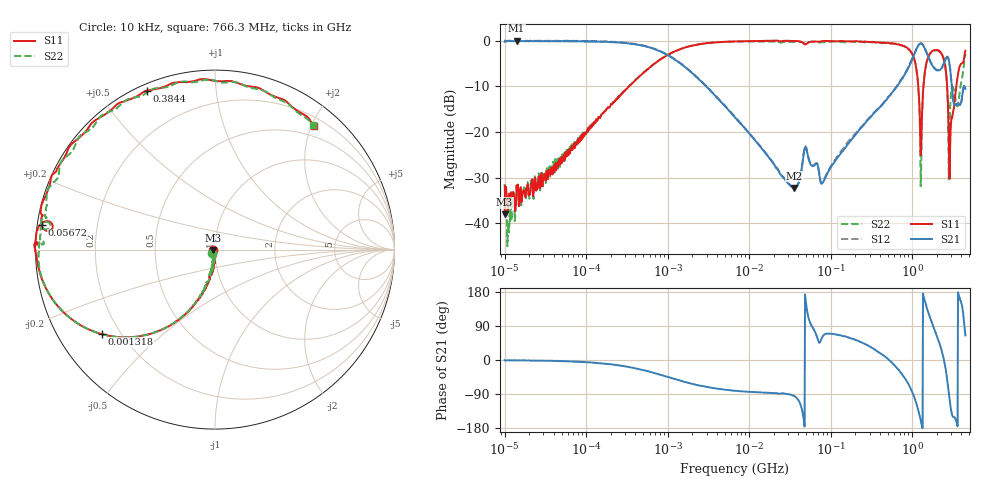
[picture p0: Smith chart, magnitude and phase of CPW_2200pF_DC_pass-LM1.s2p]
!Siglent Technologies,SNA5004A,SNA5XCED5R0097,V1.0.0.2.10.R9
!Date: 2024-10-29 17:12:58
!Data & Calibration Information:
!Freq	S11:F2(ON)	S21:F2(ON)	S12:F2(ON)	S22:F2(ON)
# Hz S DB R 50
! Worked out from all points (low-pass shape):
!   1001 points, 10 kHz to 4.5 GHz, reference 50 ohm
!   highest |S21| = 0.01 dB at 14.03 kHz (marker M1); lowest = -32.3 dB at 35.96 MHz (marker M2)
!   |S21| within 3 dB of the highest: start of sweep to 970.2 kHz; 1.058 GHz to 1.535 GHz (476.6 MHz wide, 36.8 % of centre)
!   lowest |S11| = -38.0 dB at 10 kHz (marker M3), VSWR 1.03, Z = 48.8 - j0.332 ohm
!   |S11| at or under -10 dB: start of sweep to 334.8 kHz; 1.188 GHz to 1.374 GHz (186.3 MHz wide, 14.5 % of centre); 2.684 GHz to 3.483 GHz (799.1 MHz wide, 25.9 % of centre)
!   |S22| runs from -45.0 to -0.1 dB; largest |S21 - S12| = 0.027
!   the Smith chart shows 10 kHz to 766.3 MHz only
!   S11 on the Smith chart (normalised r, x): 10 kHz: 0.98, -0.01; 1.318 MHz: 0.13, -0.33; 56.72 MHz: 0.01, +0.07; 384.4 MHz: 0.03, +0.66; 766.3 MHz: 0.33, +2.05
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10000  -38.03 -164.3  -0.18 -0.8  -0.07 -0.8  -31.47 -128.3
11390.22  -33.52 -85.5  -0.03 -0.9  0.03 -0.9  -40.75 -81.3
14027.6  -31.73 -76.8  0.01 -1.5  0.07 -1.5  -31.71 -80.3
87919.76  -21.66 -96.9  -0.12 -4.8  -0.05 -4.8  -21.43 -99.5
772988.4  -4.37 -128.4  -2.15 -37.5  -2.08 -37.4  -4.35 -128.6
1318119  -2.07 -143.3  -4.48 -52.4  -4.41 -52.4  -2.05 -143.4
6708204  -0.13 -172.7  -16.81 -81.3  -16.64 -81.3  -0.15 -172.6
3.596422e7  -0.00 174.7  -32.29 -95.5  -32.14 -95.5  -0.22 174.3
5.671959e7  -0.23 172.0  -27.08 95.8  -26.94 95.8  -0.18 171.8
5.897837e7  -0.18 171.2  -27.44 88.7  -27.30 88.6  -0.17 171.1
8.060646e7  -0.04 167.6  -31.06 63.5  -30.84 63.5  -0.30 168.0
3.843752e8  -0.32 113.2  -14.90 21.4  -14.74 21.7  -0.43 114.0
5.185364e8  -0.50 91.4  -12.21 0.3  -12.13 0.9  -0.45 92.0
7.66259e8  -1.10 51.1  -8.15 -40.6  -7.98 -39.6  -1.09 51.9
1.117683e9  -5.74 -17.5  -1.99 -112.3  -1.92 -111.7  -5.83 -20.1
1.323764e9  -15.81 78.2  -0.71 -174.5  -0.62 -173.7  -15.96 91.3
1.527552e9  -4.27 39.6  -2.88 134.4  -2.79 135.4  -4.28 45.0
1.832909e9  -2.08 -8.1  -5.80 86.5  -5.70 87.4  -2.18 -3.1
2.440684e9  -4.03 -99.1  -5.03 3.0  -4.96 4.1  -3.86 -86.6
2.966946e9  -19.44 -93.6  -7.26 -125.3  -7.21 -123.6  -12.53 -48.4
3.606682e9  -7.91 52.8  -13.85 -175.0  -13.77 -172.8  -14.39 130.9
4.5e9  -2.14 -36.9  -10.54 64.7  -10.67 61.2  -2.89 -17.8
